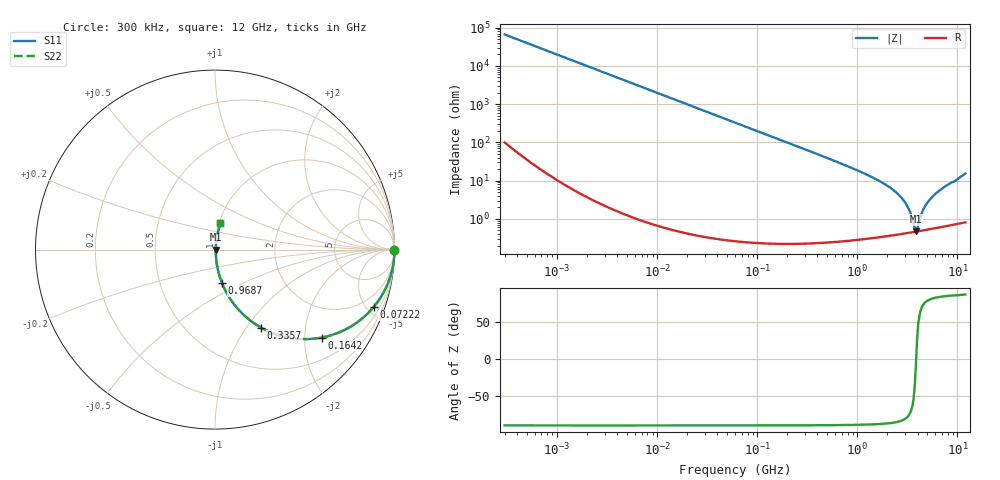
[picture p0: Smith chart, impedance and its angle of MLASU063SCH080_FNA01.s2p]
! MLASU063SCH080_FNA01  S-PARAMETER MODEL  ( Standard Model )
! Model Generated by TAIYO YUDEN Corporation (http://www.ty-top.com)
! Version 1.0
! TAIYO YUDEN Control No. 240819
! Copyright(c) 2024 TAIYO YUDEN CO.,LTD. All Rights Reserved.
! Product Description (link to TY-COMPAS)
! https://ds.yuden.co.jp/TYCOMPAS/or/detail?pn=MLASU063SCH080DFNA01&u=M
! Products Name : Multilayer Ceramic Capacitors
! Characteristics :
!  Capacitance : 8 [pF] , Rated Voltage : 50 [V] , TCC : CH / C0H
!  Case Size : 0.6 x 0.3 / 0.024 x 0.012 [mm/inch] , Thickness : 0.3 / 0.012 [mm/inch]
!  (Conditions: Temperature = 25 [degC] , DC Bias Voltage = 0 [V])
! External Node Assignments :
!  1  o---| |---o  2
! GND o---------o GND
! Frequency Range : 0.3MHz  -  12000MHz  [ 401 STEP ]
# MHZ S RI R 50
! Freq[MHz].  S11 Real  S11 Imag  S21 Real  S21 Imag  S12 Real  S12 Imag  S22 Real  S22 Imag
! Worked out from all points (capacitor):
!   401 points, 300 kHz to 12 GHz, reference 50 ohm
!   read as one part in series: C = 8 pF near 316.3 kHz
!   lowest |Z| = 470 mohm at 3.841 GHz (marker M1)
!   series resonance near 3.868 GHz, so ESL is about 210 pH
!   S11 on the Smith chart (normalised r, x): 300 kHz: open; 72.22 MHz: 1.00, -5.51; 164.2 MHz: 1.00, -2.42; 335.7 MHz: 1.00, -1.18; 968.7 MHz: 1.01, -0.38; 12 GHz: 1.02, +0.31
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0.3  1 -0.00151  4.54e-06 0.00151  4.54e-06 0.00151  1 -0.00151
1.769972  0.9999 -0.0089  8.26e-05 0.0089  8.26e-05 0.0089  0.9999 -0.0089
10.44266  0.9972 -0.0524  0.00277 0.0524  0.00277 0.0524  0.9972 -0.0524
27.10171  0.9817 -0.1338  0.0183 0.1338  0.0183 0.1338  0.9817 -0.1338
60  0.9164 -0.2764  0.0836 0.2764  0.0836 0.2764  0.9164 -0.2764
72.22496  0.8832 -0.3207  0.1168 0.3207  0.1168 0.3207  0.8832 -0.3207
164.1901  0.5937 -0.4902  0.4063 0.4902  0.4063 0.4902  0.5937 -0.4902
335.7268  0.2577 -0.4354  0.7423 0.4354  0.7423 0.4354  0.2577 -0.4354
353.9943  0.2378 -0.4237  0.7622 0.4237  0.7622 0.4237  0.2378 -0.4237
968.706  0.0382 -0.1846  0.9618 0.1846  0.9618 0.1846  0.0382 -0.1846
2088.533  0.00808 -0.0667  0.9919 0.0667  0.9919 0.0667  0.00808 -0.0667
2581.562  0.00571 -0.0424  0.9943 0.0424  0.9943 0.0424  0.00571 -0.0424
3026.31  0.00481 -0.0253  0.9952 0.0253  0.9952 0.0253  0.00481 -0.0253
3276.641  0.0046 -0.0171  0.9954 0.0171  0.9954 0.0171  0.0046 -0.0171
3642.919  0.00455 -0.00621  0.9954 0.00621  0.9954 0.00621  0.00455 -0.00621
3841.137  0.00462 -0.000749  0.9954 0.000749  0.9954 0.000749  0.00462 -0.000749
4050.141  0.00475 0.00497  0.9952 -0.00497  0.9952 -0.00497  0.00475 0.00497
4385.161  0.00506 0.0127  0.9949 -0.0127  0.9949 -0.0127  0.00506 0.0127
4747.894  0.00551 0.0207  0.9945 -0.0207  0.9945 -0.0207  0.00551 0.0207
5565.855  0.00679 0.0361  0.9932 -0.0361  0.9932 -0.0361  0.00679 0.0361
7254.098  0.0104 0.0644  0.9896 -0.0644  0.9896 -0.0644  0.0104 0.0644
12000  0.0305 0.1477  0.9695 -0.1477  0.9695 -0.1477  0.0305 0.1477
